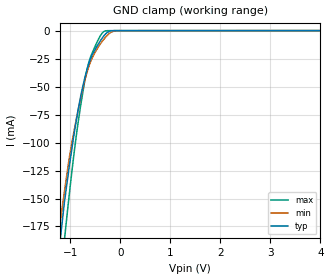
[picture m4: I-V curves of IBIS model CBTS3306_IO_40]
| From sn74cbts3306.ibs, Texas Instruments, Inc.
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[Model]   CBTS3306_IO_40
Model_type  Terminator
| variable   typ   min   max
C_comp   6pF   NA   NA
| C_tri-state   9.90pF   7.75pF   15.11pF
[Temperature Range]   40   100   -40
| Ambient temperature   25   85   -40
[Voltage range]   4   4   4
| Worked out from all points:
|   GND clamp passes 1 mA (typ) near -0.23 V on its own axis
[GND Clamp]
| CBTS3306_IO_40
|   Voltage   I(typ)   I(min)   I(max)
-4V       -2.473A    -2.423A    -2.401A
-1.245V   -206.1mA   -186.4mA   -245mA
-1.18V    -179.6mA   -165.1mA   -215.7mA
-1.115V   -153.4mA   -144.2mA   -187.2mA
-1.065V   -136.6mA   -128.4mA   -166mA
-875mV    -79.58mA   -78.65mA   -93.01mA
-795mV    -59.9mA    -61.14mA   -68.34mA
-685mV    -38.41mA   -40.63mA   -39.42mA
-565mV    -22.08mA   -24.82mA   -20.51mA
-325mV    -4.579mA   -7.588mA   -756.5uA
-55mV     -2.556uA   -50.54uA   -5.285nA
4V        3.456uA    49.22uA    47.63nA
